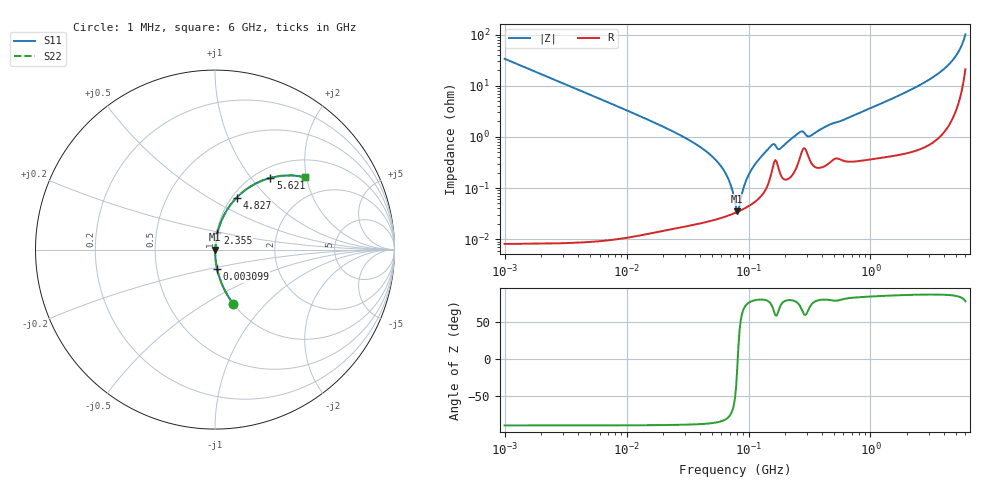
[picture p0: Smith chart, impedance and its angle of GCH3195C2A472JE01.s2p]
!Murata Part Number: GCH3195C2A472JE01
!These Parameters are Measured in Series Mode Connection
!Data Generated on Jun 19, 2026
!  o--ll--o
!Port1  Port2
!  o------o
!Operation Temp=25[degC], DC Bias Voltage=0[V]
!Freq. Start=1000[kHz] Stop=6[GHz] 401[Steps]
# Hz S RI R 50
!Freq.(Hz) S11(Real) S11(Imag) S21(Real) S21(Imag) S12(Real) S12(Imag) S22(Real) S22(Imag)
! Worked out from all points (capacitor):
!   401 points, 1 MHz to 6 GHz, reference 50 ohm
!   read as one part in series: C = 4.73 nF near 1.044 MHz
!   lowest |Z| = 34.8 mohm at 80.9 MHz (marker M1)
!   series resonance near 81.58 MHz, so ESL is about 810 pH
!   S11 on the Smith chart (normalised r, x): 1 MHz: 1.00, -0.67; 3.099 MHz: 1.00, -0.22; 2.355 GHz: 1.01, +0.19; 4.827 GHz: 1.05, +0.67; 5.621 GHz: 1.17, +1.25; 6 GHz: 1.42, +1.97
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1000000  0.1018 -0.3023  0.8982 0.3023  0.8982 0.3023  0.1018 -0.3023
3098558  0.0117 -0.1072  0.9883 0.1072  0.9883 0.1072  0.0117 -0.1072
4293785  0.00616 -0.0777  0.9938 0.0777  0.9938 0.0777  0.00616 -0.0777
1.843659e7  0.000439 -0.0173  0.9996 0.0173  0.9996 0.0173  0.000439 -0.0173
3.540316e7  0.00025 -0.0077  0.9998 0.0077  0.9998 0.0077  0.00025 -0.0077
5.236714e7  0.000252 -0.00378  0.9997 0.00378  0.9997 0.00378  0.000252 -0.00378
6.652088e7  0.000287 -0.0017  0.9997 0.0017  0.9997 0.0017  0.000287 -0.0017
7.256705e7  0.000307 -0.000976  0.9997 0.000976  0.9997 0.000976  0.000307 -0.000976
7.745967e7  0.000326 -0.000432  0.9997 0.000432  0.9997 0.000432  0.000326 -0.000432
8.090333e7  0.000341 -6.9e-05  0.9997 6.9e-05  0.9997 6.9e-05  0.000341 -6.9e-05
8.450008e7  0.000358 0.000295  0.9996 -0.000295  0.9996 -0.000295  0.000358 0.000295
9.218041e7  0.000398 0.00103  0.9996 -0.00103  0.9996 -0.00103  0.000398 0.00103
1.027698e8  0.000464 0.00198  0.9995 -0.00198  0.9995 -0.00198  0.000464 0.00198
1.520136e8  0.00177 0.00634  0.9982 -0.00634  0.9982 -0.00634  0.00177 0.00634
1.809028e8  0.00201 0.00547  0.998 -0.00547  0.998 -0.00547  0.00201 0.00547
2.675853e8  0.00449 0.0118  0.9955 -0.0118  0.9955 -0.0118  0.00449 0.0118
3.325952e8  0.00301 0.0106  0.997 -0.0106  0.997 -0.0106  0.00301 0.0106
1.428092e9  0.00685 0.0522  0.9932 -0.0522  0.9932 -0.0522  0.00685 0.0522
2.355049e9  0.0139 0.0919  0.9861 -0.0919  0.9861 -0.0919  0.0139 0.0919
4.827224e9  0.1202 0.2892  0.8798 -0.2892  0.8798 -0.2892  0.1202 0.2892
5.62102e9  0.3087 0.4  0.6913 -0.4  0.6913 -0.4  0.3087 0.4
6e9  0.5022 0.4046  0.4978 -0.4046  0.4978 -0.4046  0.5022 0.4046
